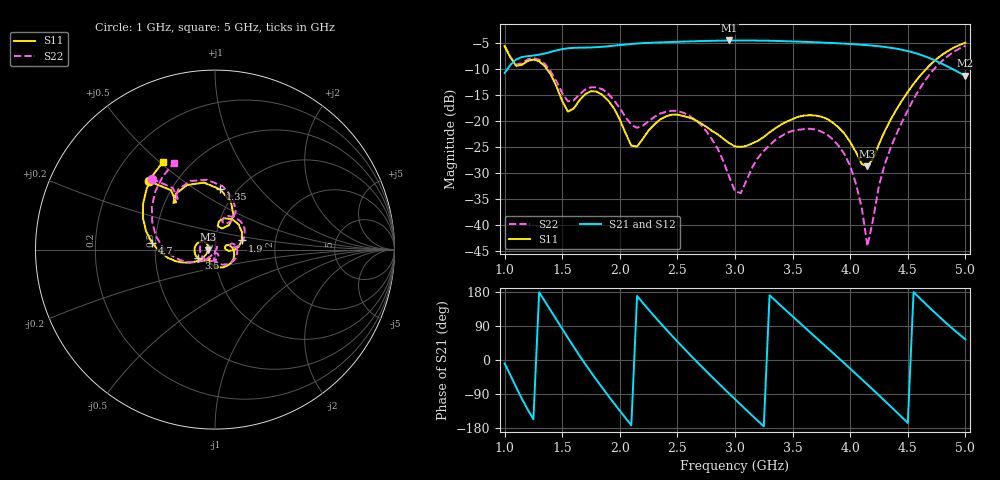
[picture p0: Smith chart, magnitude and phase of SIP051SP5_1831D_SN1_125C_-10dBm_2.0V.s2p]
# GHz  S  dB  R  50
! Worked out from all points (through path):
!   81 points, 1 GHz to 5 GHz, reference 50 ohm
!   highest |S21| = -4.46 dB at 2.95 GHz (marker M1); lowest = -11.3 dB at 5 GHz (marker M2)
!   lowest |S11| = -28.7 dB at 4.15 GHz (marker M3), VSWR 1.08, Z = 46.4 + j0.0397 ohm
!   |S11| at or under -10 dB: 1.368 GHz to 4.658 GHz (3.29 GHz wide, 109 % of centre)
!   |S22| runs from -44.0 to -5.5 dB; largest |S21 - S12| = 0.0018
!   S11 on the Smith chart (normalised r, x): 1 GHz: 0.36, +0.38; 1.35 GHz: 0.84, +0.64; 1.9 GHz: 1.34, +0.14; 3.5 GHz: 0.83, -0.08; 4.7 GHz: 0.48, +0.04; 5 GHz: 0.36, +0.52
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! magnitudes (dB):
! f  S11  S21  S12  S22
! 1 GHz  -5.5  -10.7  -10.7  -5.5
! 1.1 GHz  -9.3  -8.1  -8.1  -9.1
! 1.35 GHz  -9.4  -7.0  -6.9  -9.0
! 1.55 GHz  -18.1  -6.0  -6.0  -16.2
! 1.7 GHz  -14.8  -5.8  -5.8  -13.9
! 1.9 GHz  -16.0  -5.6  -5.6  -14.7
! 2.1 GHz  -24.7  -5.1  -5.1  -20.7
! 2.35 GHz  -19.6  -4.8  -4.8  -18.5
! 2.7 GHz  -20.3  -4.6  -4.6  -20.6
! 2.95 GHz  -24.2  -4.5  -4.5  -30.7
! 3 GHz  -24.8  -4.5  -4.5  -33.5
! 3.05 GHz  -24.9  -4.5  -4.5  -33.8
! 3.25 GHz  -23.0  -4.5  -4.5  -25.7
! 3.5 GHz  -19.6  -4.7  -4.6  -21.8
! 3.7 GHz  -18.9  -4.8  -4.8  -21.6
! 4 GHz  -24.0  -5.1  -5.1  -28.6
! 4.1 GHz  -28.2  -5.3  -5.3  -36.6
! 4.15 GHz  -28.7  -5.4  -5.4  -44.0
! 4.25 GHz  -24.4  -5.6  -5.6  -32.3
! 4.35 GHz  -19.7  -5.9  -5.9  -25.2
! 4.7 GHz  -9.0  -7.9  -8.0  -10.7
! 5 GHz  -4.9  -11.3  -11.3  -5.5
